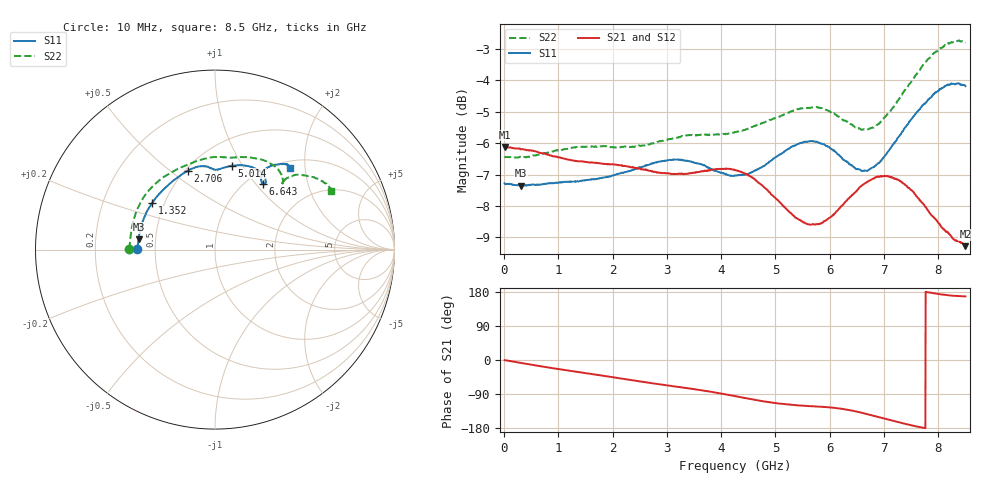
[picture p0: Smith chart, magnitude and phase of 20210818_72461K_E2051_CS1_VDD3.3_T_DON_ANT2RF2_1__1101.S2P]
!Agilent Technologies,E5071C,MY46417908,A.11.23
!Date: Wed Aug 18 14:27:35 2021
!Data & Calibration Information:
!Freq	S11:SOLT2(ON)	S21:SOLT2(ON)	S12:SOLT2(ON)	S22:SOLT2(ON)
!PortZ  Port1:50+j0  Port2:50+j0
!Above PortZ is port z conversion or system Z0 setting when saving the data.
!When reading, reference impedance value at option line is always used.
# Hz S dB R 50
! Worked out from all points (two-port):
!   1601 points, 10 MHz to 8.5 GHz, reference 50 ohm
!   highest |S21| = -6.12 dB at 10 MHz (marker M1); lowest = -9.3 dB at 8.5 GHz (marker M2)
!   |S21| within 3 dB of the highest: start of sweep to 8.354 GHz; 8.365131 GHz to 8.371864 GHz (6.733 MHz wide, 0.0805 % of centre)
!   lowest |S11| = -7.4 dB at 312.5 MHz (marker M3), VSWR 2.50, Z = 20.1 + j2.8 ohm
!   |S11| at or under -10 dB: nowhere
!   |S22| runs from -6.5 to -2.7 dB; largest |S21 - S12| = 0.0016
!   S11 on the Smith chart (normalised r, x): 10 MHz: 0.40, +0.00; 1.352 GHz: 0.43, +0.27; 2.706 GHz: 0.52, +0.58; 5.014 GHz: 0.74, +0.90; 6.643 GHz: 1.18, +1.09; 8.5 GHz: 1.12, +1.66
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1e7  -7.28 179.6  -6.12 -0.4  -6.12 -0.4  -6.42 179.6
3.124562e8  -7.36 172.4  -6.20 -7.8  -6.18 -7.8  -6.45 171.4
9.279812e8  -7.27 156.2  -6.42 -22.3  -6.42 -22.2  -6.25 153.9
1.352481e9  -7.21 143.5  -6.57 -31.4  -6.57 -31.4  -6.12 141.0
1.426769e9  -7.20 141.2  -6.58 -33.0  -6.58 -32.9  -6.11 138.7
2.079438e9  -6.99 122.8  -6.69 -47.1  -6.70 -47.1  -6.14 119.6
2.705575e9  -6.65 109.1  -6.88 -61.0  -6.88 -61.0  -6.02 104.3
2.843538e9  -6.60 106.8  -6.93 -63.7  -6.93 -63.7  -5.95 101.5
3.384775e9  -6.57 98.3  -6.97 -74.6  -6.96 -74.6  -5.75 91.2
4.255e9  -7.03 89.3  -6.86 -95.4  -6.85 -95.4  -5.65 79.3
4.674194e9  -6.84 85.0  -7.24 -106.5  -7.23 -106.5  -5.42 74.1
5.013794e9  -6.44 78.8  -7.77 -113.9  -7.78 -113.8  -5.19 68.7
5.321556e9  -6.10 71.4  -8.30 -118.7  -8.30 -118.6  -4.97 62.8
5.671769e9  -5.94 62.6  -8.59 -122.0  -8.60 -122.0  -4.87 55.8
6.08035e9  -6.22 54.8  -8.25 -126.2  -8.27 -126.3  -5.05 48.5
6.361581e9  -6.67 52.8  -7.75 -132.2  -7.76 -132.3  -5.38 45.2
6.642812e9  -6.88 54.0  -7.29 -141.1  -7.29 -141.2  -5.56 44.4
7.088538e9  -6.23 57.9  -7.06 -157.8  -7.08 -157.9  -5.04 45.0
7.422831e9  -5.43 57.8  -7.37 -169.5  -7.37 -169.6  -4.22 42.7
7.8208e9  -4.61 53.8  -8.17 178.5  -8.15 178.4  -3.31 36.2
8.197544e9  -4.14 49.9  -8.89 170.6  -8.87 170.7  -2.83 30.0
8.5e9  -4.18 47.7  -9.28 167.8  -9.26 167.7  -2.80 26.7
